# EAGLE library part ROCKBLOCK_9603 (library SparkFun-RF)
Designed to work with SMD connector 53398-1071 from Molex.
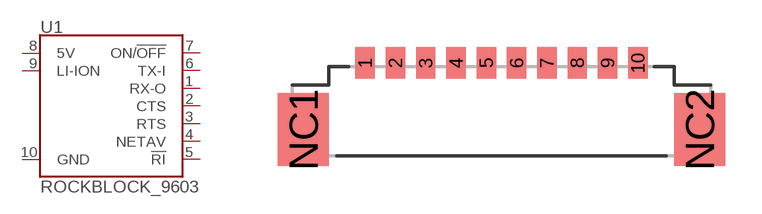
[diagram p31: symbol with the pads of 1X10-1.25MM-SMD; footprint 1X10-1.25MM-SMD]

Designator prefix U1

## ROCKBLOCK_9603SMD (PROD_ID: CONN-14655)  [1X10-1.25MM-SMD]
1  RX-O  out
2  CTS  out
3  RTS  in
4  NETAV
5  !RI!
6  TX-I
7  ON/!OFF!
8  5V
9  LI-ION
10  GND

## Footprint 1X10-1.25MM-SMD (pad centres in mm)
smd 0.8 x 1.3: 1 -5.625,2.75; 2 -4.375,2.75; 3 -3.125,2.75; 4 -1.875,2.75; 5 -0.625,2.75; 6 0.625,2.75; 7 1.875,2.75; 8 3.125,2.75; 9 4.375,2.75; 10 5.625,2.75
smd 2.1 x 3: NC1 -8.175,0; NC2 8.175,0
